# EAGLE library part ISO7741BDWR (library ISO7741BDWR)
Digital Isolators Robust EMC, quad-channel, 3/1, reinforced digital isolator 16-SOIC -55 to 125 Source: Datasheet
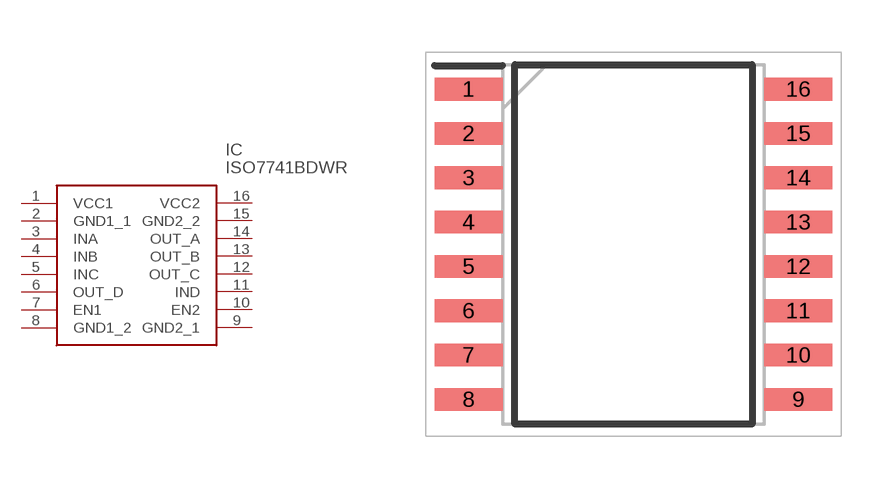
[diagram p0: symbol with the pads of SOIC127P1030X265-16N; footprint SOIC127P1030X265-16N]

Designator prefix IC

## ISO7741BDWR (Description: Digital Isolators Robust EMC, quad-channel, 3/1, reinforced digital isolator 16-SOIC -55 to 125; Height: 2.65mm; Manufacturer_Name: Texas Instruments; Manufacturer_Part_Number: ISO7741BDWR; Mouser_Part_Number: 595-ISO7741BDWR; Mouser_Price-Stock: https://www.mouser.co.uk/ProductDetail/Texas-Instruments/ISO7741BDWR?qs=OlC7AqGiEDldKlKXjTOIyw%3D%3D)  [SOIC127P1030X265-16N]
1  VCC1
2  GND1_1
3  INA
4  INB
5  INC
6  OUT_D
7  EN1
8  GND1_2
9  GND2_1
10  EN2
11  IND
12  OUT_C
13  OUT_B
14  OUT_A
15  GND2_2
16  VCC2

## Footprint SOIC127P1030X265-16N (pad centres in mm)
DW (R-PDSO-G16)
smd 1.95 x 0.65: 1 -4.725,4.445; 2 -4.725,3.175; 3 -4.725,1.905; 4 -4.725,0.635; 5 -4.725,-0.635; 6 -4.725,-1.905; 7 -4.725,-3.175; 8 -4.725,-4.445; 9 4.725,-4.445; 10 4.725,-3.175; 11 4.725,-1.905; 12 4.725,-0.635; 13 4.725,0.635; 14 4.725,1.905; 15 4.725,3.175; 16 4.725,4.445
